FUNCTION F_SlopeIntercept : LREAL	// 使用直线的斜截式方程
VAR_INPUT
    k:				LREAL;  // 斜率
    b:				LREAL;  // 截距
    x0, y0:			LREAL;  // 点坐标
END_VAR
VAR
    Numerator:		LREAL;	// 分子
    Denominator:	LREAL;	// 分母
END_VAR

// 转换为一般式：y = kx + b -> kx - y + b = 0

// 计算分子：|k*x0 - y0 + b|
Numerator := ABS(k * x0 - y0 + b);

// 计算分母：sqrt(k² + 1)
Denominator := SQRT(k * k + 1);

// 避免除零错误
IF Denominator = 0 THEN
    F_SlopeIntercept := 0.0;
ELSE
    F_SlopeIntercept := Numerator / Denominator;
END_IF

END_FUNCTION
